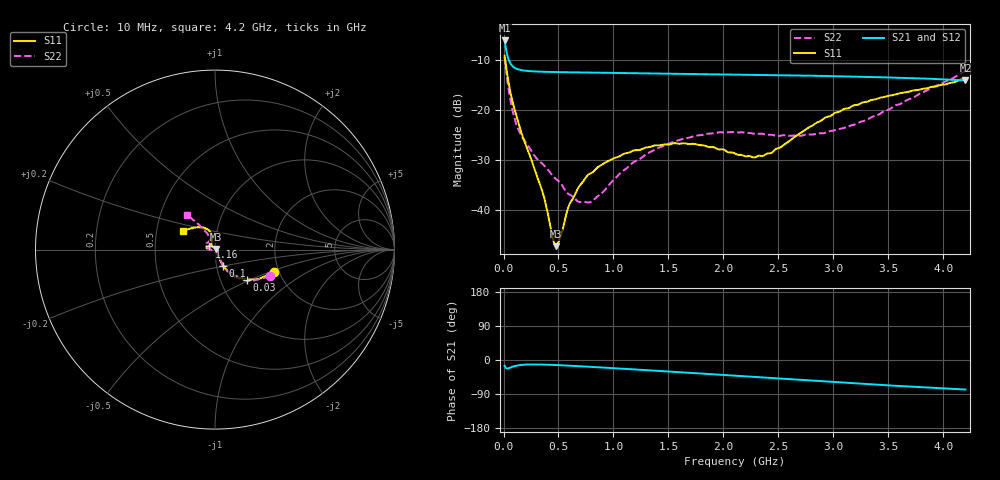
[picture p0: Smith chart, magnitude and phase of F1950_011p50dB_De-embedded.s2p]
! Integrated Device Technology
! Corporate Headquarters
! 6024 Silver Creek Valley Road
! San Jose, CA 95138  USA
! Phone:  1-408-284-8200
! Toll Free:  1-800-223-1366
! Webpage:  http://www.idt.com/
! Timing and RF Division
! 515 Groton Road, Suite 102
! Westford, MA 01886-6024
! Device:  F1950
! Description: 7-bit 0.25 dB Digital Step Attenuator
! Frequency:  150.0 -  4000.00 MHz
! Package:  4x4 mm Thin QFN Plastic Package: 24 pin
! Ports:  2 RF, 12 DC
!  Pin  1  = D0
!  Pin  2  = VDD
!  Pin  3  = Vmode
!  Pin  4  = GND
!  Pin  5  = RF1  =  Port 1
!  Pin  6  = GND
!  Pin  7  = GND
!  Pin  8  = GND
!  Pin  9  = GND
!  Pin 10  = GND
!  Pin 11  = GND
!  Pin 12  = GND
!  Pin 13  = GND
!  Pin 14  = RF2  =  Port 2
!  Pin 15  = GND
!  Pin 16  = LE
!  Pin 17  = CLK
!  Pin 18  = DATE
!  Pin 19  = D6
!  Pin 20  = D5
!  Pin 21  = D4
!  Pin 22  = D3
!  Pin 23  = D2
!  Pin 24  = D1
! State:  46
! Atten State:  11.50 dB
! Voltage:  +5.00 Volts
! Current:  Not Measured mA
! Data:  The device was measured on a the F195X evaluation board which has
!  individual transmission lines to the RF pins.  Data was collected
!  using a calibrated network analyzer.  The evaluation board was
!  de-embedded using a TRL calibration technique.
!  The reference plane is the edge of the package pin.
! Misc:  Board 2019
!  Action Tracker AT0250
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# GHz S dB R 50
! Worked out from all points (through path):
!   420 points, 10 MHz to 4.2 GHz, reference 50 ohm
!   highest |S21| = -6.05 dB at 10 MHz (marker M1); lowest = -14.0 dB at 4.2 GHz (marker M2)
!   group delay of S21, straight-line fit = 47.4 ps
!   lowest |S11| = -47.2 dB at 480 MHz (marker M3), VSWR 1.01, Z = 50.3 + j0.281 ohm
!   |S11| at or under -10 dB: 15.69 MHz to end of sweep
!   |S22| runs from -38.5 to -9.4 dB; largest |S21 - S12| = 0.00032
!   S11 on the Smith chart (normalised r, x): 10 MHz: 1.87, -0.54; 30 MHz: 1.34, -0.48; 100 MHz: 1.08, -0.20; 1.16 GHz: 0.93, +0.03; 4.2 GHz: 0.68, +0.15
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0.01  -9.09 -21.1  -6.05 -15.3  -6.04 -15.3  -9.36 -26.0
0.03  -12.21 -42.8  -8.56 -22.4  -8.56 -22.4  -13.27 -49.6
0.06  -16.13 -56.6  -10.53 -20.2  -10.53 -20.2  -17.60 -60.6
0.1  -19.79 -63.5  -11.49 -16.1  -11.49 -16.1  -21.60 -62.2
0.15  -23.61 -64.3  -11.92 -13.4  -11.92 -13.4  -24.56 -63.1
0.27  -30.96 -56.8  -12.22 -11.7  -12.22 -11.7  -28.70 -63.4
0.37  -37.47 -41.0  -12.31 -12.1  -12.31 -12.1  -31.06 -65.5
0.45  -45.77 -1.8  -12.35 -12.9  -12.35 -13.0  -33.18 -69.2
0.48  -47.16 39.5  -12.37 -13.3  -12.37 -13.3  -33.79 -72.9
0.52  -45.06 81.8  -12.38 -13.8  -12.38 -13.8  -34.57 -74.7
0.6  -38.77 111.7  -12.41 -15.0  -12.41 -15.0  -36.86 -88.0
0.71  -34.63 124.7  -12.44 -16.7  -12.44 -16.7  -38.36 -111.7
0.81  -32.39 132.0  -12.47 -18.3  -12.47 -18.4  -38.10 -139.8
1.16  -28.25 152.8  -12.58 -24.3  -12.58 -24.3  -30.76 175.0
1.41  -27.00 164.7  -12.65 -28.8  -12.65 -28.8  -27.49 166.0
1.73  -26.71 172.8  -12.74 -34.5  -12.73 -34.5  -25.17 157.6
2.11  -28.72 163.4  -12.85 -41.5  -12.85 -41.6  -24.43 147.7
2.43  -28.57 125.7  -12.96 -47.3  -12.96 -47.3  -24.91 136.9
2.81  -23.04 103.0  -13.10 -54.4  -13.09 -54.5  -24.85 120.6
3.1  -19.70 106.0  -13.22 -59.8  -13.22 -59.9  -23.52 115.1
3.51  -17.06 118.3  -13.44 -67.1  -13.44 -67.2  -19.80 116.4
4.2  -13.61 149.6  -14.04 -77.9  -14.03 -78.0  -12.15 128.6
